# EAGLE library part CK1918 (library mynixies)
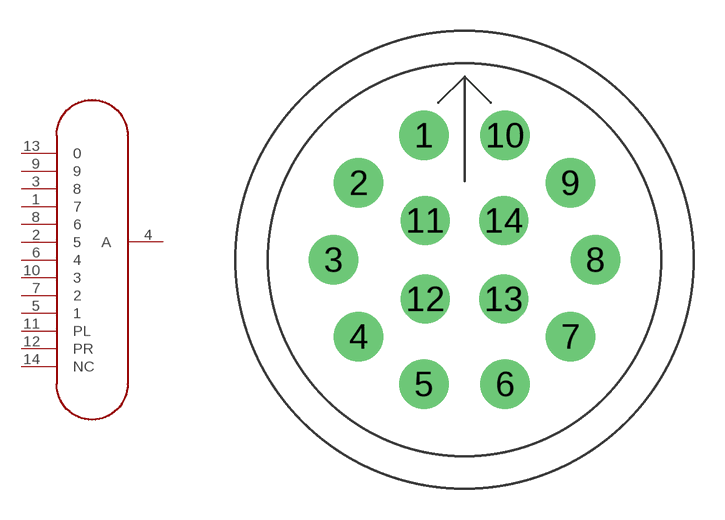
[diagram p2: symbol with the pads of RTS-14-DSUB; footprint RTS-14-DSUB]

Designator prefix U

## CK1918  [RTS-14-DSUB]
1  7  pas
2  5  pas
3  8  pas
4  A  pas
5  1  pas
6  4  pas
7  2  pas
8  6  pas
9  9  pas
10  3  pas
11  PL  pas
12  PR  pas
13  0  pas
14  NC  nc

## Footprint RTS-14-DSUB (pad centres in mm)
drill 1.6: 1 -1.962,6.039; 2 -5.137,3.732; 3 -6.35,0; 4 -5.137,-3.732; 5 -1.962,-6.039; 6 1.962,-6.039; 7 5.137,-3.732; 8 6.35,0; 9 5.137,3.732; 10 1.962,6.039; 11 -1.904,1.904; 12 -1.904,-1.904; 13 1.904,-1.904; 14 1.904,1.904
